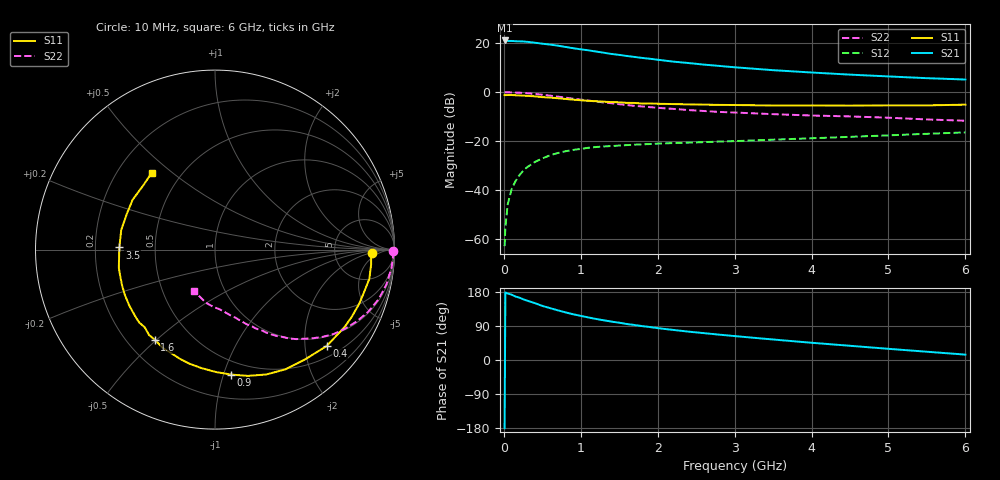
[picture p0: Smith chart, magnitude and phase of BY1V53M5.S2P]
! SIEMENS Small Signal Semiconductors
! BFY420
! Si NPN RF SIEGET Grounded Emitter Transistor in MICRO-X
! VCE = 1.5 V  IC = 3.5 mA
! Common Emitter S-Parameters:  October  1996
# GHz  S  MA  R  50
!  f  S11  S21  S12  S22
! GHz  MAG  ANG  MAG  ANG  MAG  ANG  MAG  ANG
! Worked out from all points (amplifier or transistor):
!   36 points, 10 MHz to 6 GHz, reference 50 ohm
!   highest |S21| = 21.2 dB at 10 MHz (marker M1)
!   |S21| within 3 dB of that: start of sweep to 867 MHz
!   unconditionally stable (mu >= 1): 3.434 GHz to end of sweep
!   at 250 MHz: K = 0.08, MSG = 26.5 dB, |S12| = -32.3 dB
!   at 1.4 GHz: K = 0.43, MSG = 18.9 dB, |S12| = -22.1 dB
!   at 6 GHz: K = 1.18, MAG = 8.2 dB, |S12| = -16.5 dB
!   S11 on the Smith chart (normalised r, x): 10 MHz: 14, -3; 400 MHz: 0.75, -2.49; 900 MHz: 0.39, -1.06; 1.6 GHz: 0.31, -0.49; 3.5 GHz: 0.30, +0.01; 6 GHz: 0.34, +0.43
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0.01  0.8727 -1.4  11.46 -179.9  0.0007 91.6  0.9939 -0.6
0.02  0.8706 -2.4  11.42 178.1  0.0017 83.0  0.9909 -1.0
0.05  0.8738 -5.4  11.19 175.5  0.005 89.6  0.9923 -2.8
0.1  0.8752 -10.7  11.2 172.5  0.0102 87.1  0.9886 -5.8
0.15  0.8639 -15.8  11.05 167.6  0.0149 79.9  0.9806 -8.7
0.25  0.8488 -26.4  10.94 160.4  0.0244 75.3  0.9628 -14.2
0.3  0.8406 -31.0  10.76 156.7  0.0288 73.0  0.9521 -17.0
0.4  0.822 -40.8  10.33 150.3  0.0369 67.3  0.9211 -22.1
0.5  0.7915 -50.5  9.821 142.8  0.0439 63.0  0.886 -26.8
0.6  0.7742 -59.5  9.452 137.0  0.0509 58.8  0.8483 -31.3
0.7  0.752 -67.7  8.973 131.2  0.0566 55.0  0.8116 -35.4
0.9  0.7022 -82.6  7.955 120.7  0.0657 47.8  0.7374 -42.0
1.1  0.6646 -96.5  7.192 112.2  0.0726 42.9  0.6732 -47.8
1.4  0.626 -113.3  6.059 101.3  0.0787 37.0  0.5925 -54.4
1.6  0.6036 -123.7  5.504 94.9  0.0823 34.1  0.5451 -58.2
2  0.5793 -140.1  4.616 84.1  0.0883 30.3  0.4772 -64.0
2.2  0.5702 -146.9  4.231 79.4  0.0905 29.0  0.4547 -66.7
2.8  0.5483 -164.4  3.45 66.9  0.0972 26.4  0.3938 -73.6
3.5  0.5331 178.7  2.822 54.1  0.1064 24.5  0.3544 -80.7
4.5  0.5301 158.0  2.286 37.5  0.1216 21.4  0.3186 -91.9
5.5  0.5361 138.4  1.934 21.8  0.1403 17.3  0.2762 -107.6
6  0.5548 129.4  1.816 14.2  0.15 14.6  0.2599 -117.1
